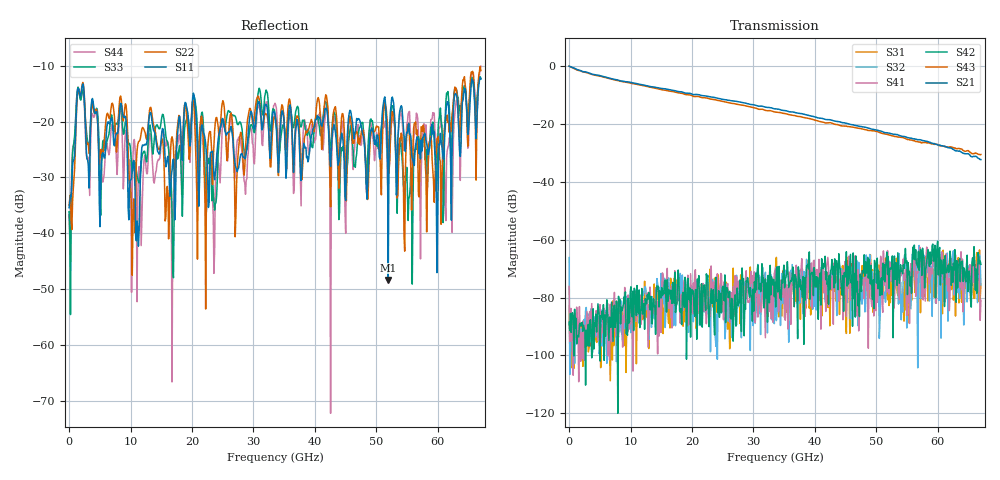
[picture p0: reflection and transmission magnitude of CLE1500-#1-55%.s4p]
!Keysight Technologies,N5247B,US50470101,A.16.20.02
!Date: Thursday, March 13, 2025 10:24:06
!Correction: S11(C  4-Port  )
!S12(C  4-Port  )
!S13(C  4-Port  )
!S14(C  4-Port  )
!S21(C  4-Port  )
!S22(C  4-Port  )
!S23(C  4-Port  )
!S24(C  4-Port  )
!S31(C  4-Port  )
!S32(C  4-Port  )
!S33(C  4-Port  )
!S34(C  4-Port  )
!S41(C  4-Port  )
!S42(C  4-Port  )
!S43(C  4-Port  )
!S44(C  4-Port  )
!S4P File: Measurements: <S11,S12,S13,S14>,
!<S21,S22,S23,S24>,
!<S31,S32,S33,S34>,
!<S41,S42,S43,S44>:
# Hz S  dB  R 50
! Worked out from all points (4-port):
!   601 points, 10 MHz to 67 GHz, reference 50 ohm
!   strongest paths, dB at 10 MHz, 16.76 GHz, 33.51 GHz, 50.25 GHz, 67 GHz:
!     S21: 0.0, -8.3, -14.8, -22.2, -32.3
!     S43: 0.0, -8.7, -15.8, -22.7, -30.5
!     S42: -88.5, -82.1, -74.7, -76.9, -68.5
!     S41: -76.1, -90.5, -70.7, -77.1, -80.9
!     S32: -66.2, -75.3, -71.3, -70.2, -75.6
!     S31: -83.0, -81.1, -75.0, -72.4, -75.3
!   lowest |S11| = -48.3 dB at 51.93 GHz (marker M1), VSWR 1.01, Z = 50 + j0.381 ohm
!   |S11| at or under -10 dB: start of sweep to end of sweep
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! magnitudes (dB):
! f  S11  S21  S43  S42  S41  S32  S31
! 10 MHz  -35.4  0.0  0.0  -88.5  -76.1  -66.2  -83.0
! 1.573 GHz  -14.2  -1.3  -1.5  -93.6  -109.1  -90.8  -92.2
! 11.18 GHz  -39.1  -6.1  -6.4  -83.1  -80.4  -82.1  -84.6
! 20.33 GHz  -15.2  -9.8  -10.5  -84.4  -80.1  -80.3  -81.1
! 23.57 GHz  -29.6  -10.8  -11.5  -87.8  -80.8  -75.6  -83.5
! 51.93 GHz  -48.3  -23.1  -23.7  -65.8  -73.5  -75.5  -75.1
! 67 GHz  -12.4  -32.3  -30.5  -68.5  -80.9  -75.6  -75.3
